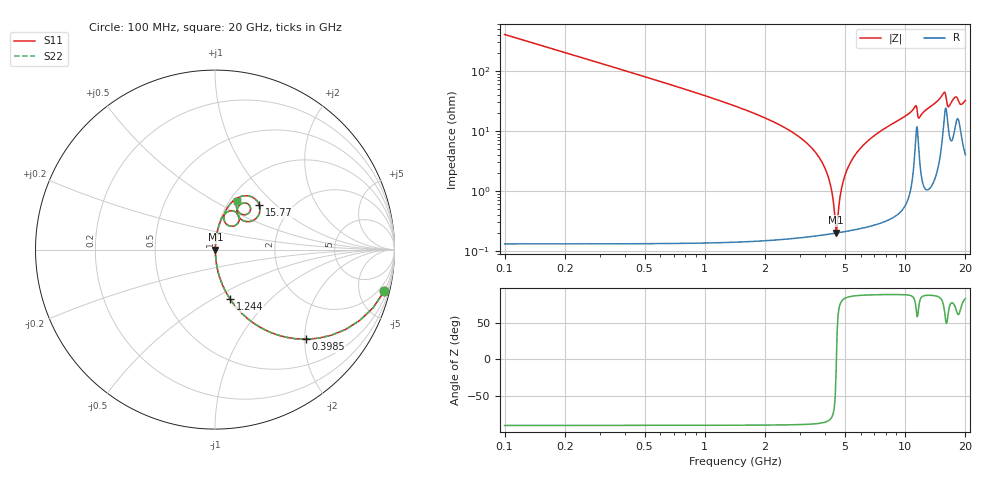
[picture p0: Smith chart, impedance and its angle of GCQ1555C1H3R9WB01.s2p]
!Murata Part Number: GCQ1555C1H3R9WB01
!These Parameters are Measured in Series Mode Connection
!Data Generated on Mar 13, 2026
!  o--ll--o
!Port1  Port2
!  o------o
!Operation Temp=25[degC], DC Bias Voltage=0[V]
!Freq. Start=100[MHz] Stop=20[GHz] 401[Steps]
# Hz S RI R 50
!Freq.(Hz) S11(Real) S11(Imag) S21(Real) S21(Imag) S12(Real) S12(Imag) S22(Real) S22(Imag)
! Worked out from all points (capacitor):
!   401 points, 100 MHz to 20 GHz, reference 50 ohm
!   read as one part in series: C = 3.9 pF near 199.5 MHz
!   lowest |Z| = 202 mohm at 4.528 GHz (marker M1)
!   series resonance near 4.538 GHz, so ESL is about 320 pH
!   S11 on the Smith chart (normalised r, x): 100 MHz: 1.00, -8.16; 398.5 MHz: 1.00, -2.03; 1.244 GHz: 1.00, -0.61; 15.77 GHz: 1.40, +0.79; 20 GHz: 1.08, +0.64
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1e8  0.9432 -0.2312  0.0568 0.2312  0.0568 0.2312  0.9432 -0.2312
3.985e8  0.508 -0.4993  0.492 0.4993  0.492 0.4993  0.508 -0.4993
7.4675e8  0.221 -0.4137  0.779 0.4137  0.779 0.4137  0.221 -0.4137
1.24425e9  0.0854 -0.2772  0.9146 0.2772  0.9146 0.2772  0.0854 -0.2772
3.43325e9  0.00432 -0.0508  0.9957 0.0508  0.9957 0.0508  0.00432 -0.0508
4.12975e9  0.00217 -0.017  0.9978 0.017  0.9978 0.017  0.00217 -0.017
4.52775e9  0.00197 -0.000401  0.998 0.000401  0.998 0.000401  0.00197 -0.000401
4.62725e9  0.00201 0.00354  0.998 -0.00354  0.998 -0.00354  0.00201 0.00354
4.876e9  0.00222 0.0131  0.9978 -0.0131  0.9978 -0.0131  0.00222 0.0131
5.22425e9  0.0028 0.0257  0.9972 -0.0257  0.9972 -0.0257  0.0028 0.0257
5.82125e9  0.00441 0.0459  0.9956 -0.0459  0.9956 -0.0459  0.00441 0.0459
6.7665e9  0.00828 0.0752  0.9917 -0.0752  0.9917 -0.0752  0.00828 0.0752
1.005e10  0.036 0.1707  0.964 -0.1707  0.964 -0.1707  0.036 0.1707
1.1244e10  0.106 0.2139  0.894 -0.2139  0.894 -0.2139  0.106 0.2139
1.17415e10  0.0626 0.1428  0.9374 -0.1428  0.9374 -0.1428  0.0626 0.1428
1.338325e10  0.0704 0.2346  0.9296 -0.2346  0.9296 -0.2346  0.0704 0.2346
1.577125e10  0.2472 0.2482  0.7528 -0.2482  0.7528 -0.2482  0.2472 0.2482
1.63185e10  0.1538 0.1629  0.8462 -0.1629  0.8462 -0.1629  0.1538 0.1629
1.67165e10  0.1225 0.2119  0.8775 -0.2119  0.8775 -0.2119  0.1225 0.2119
1.77115e10  0.1776 0.2574  0.8224 -0.2574  0.8224 -0.2574  0.1776 0.2574
1.89055e10  0.1407 0.2013  0.8593 -0.2013  0.8593 -0.2013  0.1407 0.2013
2e10  0.1224 0.2713  0.8776 -0.2713  0.8776 -0.2713  0.1224 0.2713
